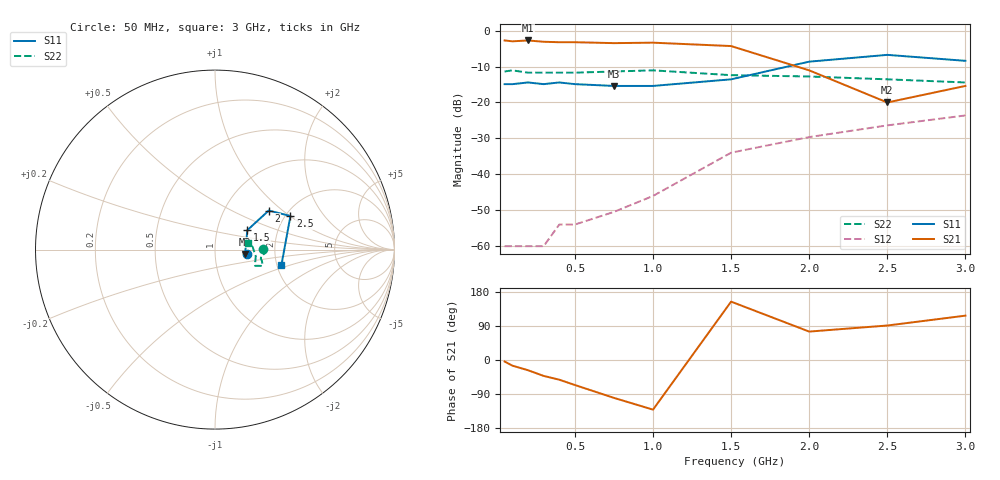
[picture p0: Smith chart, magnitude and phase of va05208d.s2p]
!  IVA-05208  S PARAMETERS
!  S PARAMETERS (VGC=5.0V, Id=32.3mA)!  LAST UPDATED 08-11-93
# ghz s ma r 50
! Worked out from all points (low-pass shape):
!   12 points, 50 MHz to 3 GHz, reference 50 ohm
!   highest |S21| = -2.73 dB at 200 MHz (marker M1); lowest = -20.0 dB at 2.5 GHz (marker M2)
!   |S21| within 3 dB of the highest: start of sweep to 1.606 GHz
!   lowest |S11| = -15.4 dB at 750 MHz (marker M3), VSWR 1.41, Z = 70.1 - j3.42 ohm
!   |S11| at or under -10 dB: start of sweep to 1.861 GHz
!   |S22| runs from -14.4 to -11.1 dB; largest |S21 - S12| = 0.73
!   S11 on the Smith chart (normalised r, x): 50 MHz: 1.43, -0.06; 1.5 GHz: 1.40, +0.32; 2 GHz: 1.60, +0.81; 2.5 GHz: 2.12, +1.01; 3 GHz: 2.12, -0.42
0.05  0.18 -7.0  0.73 -4.0  0.001 78.0  0.27 1.0
0.1  0.18 -7.0  0.71 -15.0  0.001 35.0  0.28 -4.0
0.2  0.19 -7.0  0.73 -27.0  0.001 73.0  0.26 -8.0
0.3  0.18 -8.0  0.7 -42.0  0.001 103.0  0.26 -9.0
0.4  0.19 -9.0  0.69 -52.0  0.002 100.0  0.26 -10.0
0.5  0.18 -10.0  0.69 -66.0  0.002 103.0  0.26 -11.0
0.75  0.17 -8.0  0.67 -100.0  0.003 123.0  0.27 -14.0
1  0.17 1.0  0.68 -131.0  0.005 149.0  0.28 -19.0
1.5  0.21 31.0  0.61 154.0  0.02 148.0  0.24 -22.0
2  0.37 36.0  0.28 75.0  0.033 125.0  0.23 -9.0
2.5  0.46 24.0  0.1 91.0  0.048 129.0  0.21 4.0
3  0.38 -13.0  0.17 117.0  0.066 114.0  0.19 11.0
